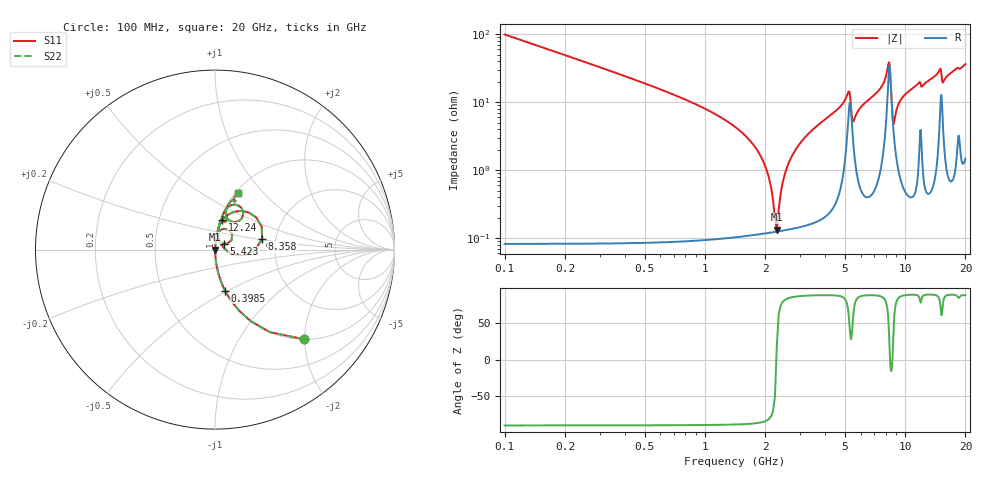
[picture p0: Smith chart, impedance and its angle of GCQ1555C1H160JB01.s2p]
!Murata Part Number: GCQ1555C1H160JB01
!These Parameters are Measured in Series Mode Connection
!Data Generated on Jan 08, 2026
!  o--ll--o
!Port1  Port2
!  o------o
!Operation Temp=25[degC], DC Bias Voltage=0[V]
!Freq. Start=100[MHz] Stop=20[GHz] 401[Steps]
# Hz S RI R 50
!Freq.(Hz) S11(Real) S11(Imag) S21(Real) S21(Imag) S12(Real) S12(Imag) S22(Real) S22(Imag)
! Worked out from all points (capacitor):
!   401 points, 100 MHz to 20 GHz, reference 50 ohm
!   read as one part in series: C = 16 pF near 199.5 MHz
!   lowest |Z| = 133 mohm at 2.289 GHz (marker M1)
!   series resonance near 2.277 GHz, so ESL is about 310 pH
!   S11 on the Smith chart (normalised r, x): 100 MHz: 1.00, -1.99; 398.5 MHz: 1.00, -0.48; 5.423 GHz: 1.10, +0.07; 8.358 GHz: 1.69, +0.22; 12.24 GHz: 1.02, +0.35; 20 GHz: 1.03, +0.73
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1e8  0.4964 -0.4996  0.5036 0.4996  0.5036 0.4996  0.4964 -0.4996
3.985e8  0.056 -0.2283  0.944 0.2283  0.944 0.2283  0.056 -0.2283
1.7915e9  0.00157 -0.0213  0.9984 0.0213  0.9984 0.0213  0.00157 -0.0213
1.9905e9  0.00131 -0.0119  0.9987 0.0119  0.9987 0.0119  0.00131 -0.0119
2.1895e9  0.00123 -0.00346  0.9988 0.00346  0.9988 0.00346  0.00123 -0.00346
2.289e9  0.00124 0.000465  0.9988 -0.000465  0.9988 -0.000465  0.00124 0.000465
2.687e9  0.00157 0.0148  0.9984 -0.0148  0.9984 -0.0148  0.00157 0.0148
3.43325e9  0.00312 0.0385  0.9969 -0.0385  0.9969 -0.0385  0.00312 0.0385
5.1745e9  0.0569 0.1155  0.9431 -0.1155  0.9431 -0.1155  0.0569 0.1155
5.42325e9  0.0477 0.0319  0.9523 -0.0319  0.9523 -0.0319  0.0477 0.0319
5.5725e9  0.0198 0.0509  0.9802 -0.0509  0.9802 -0.0509  0.0198 0.0509
6.7665e9  0.0174 0.1139  0.9826 -0.1139  0.9826 -0.1139  0.0174 0.1139
8.10975e9  0.1259 0.2141  0.8741 -0.2141  0.8741 -0.2141  0.1259 0.2141
8.3585e9  0.2618 0.0596  0.7382 -0.0596  0.7382 -0.0596  0.2618 0.0596
8.7565e9  0.0362 0.0281  0.9638 -0.0281  0.9638 -0.0281  0.0362 0.0281
1.005e10  0.0215 0.1282  0.9785 -0.1282  0.9785 -0.1282  0.0215 0.1282
1.2239e10  0.0394 0.1661  0.9606 -0.1661  0.9606 -0.1661  0.0394 0.1661
1.338325e10  0.0487 0.2047  0.9513 -0.2047  0.9513 -0.2047  0.0487 0.2047
1.49255e10  0.128 0.2463  0.872 -0.2463  0.872 -0.2463  0.128 0.2463
1.5423e10  0.0787 0.1639  0.9213 -0.1639  0.9213 -0.1639  0.0787 0.1639
1.67165e10  0.0699 0.2421  0.9301 -0.2421  0.9301 -0.2421  0.0699 0.2421
2e10  0.1267 0.3129  0.8733 -0.3129  0.8733 -0.3129  0.1267 0.3129
